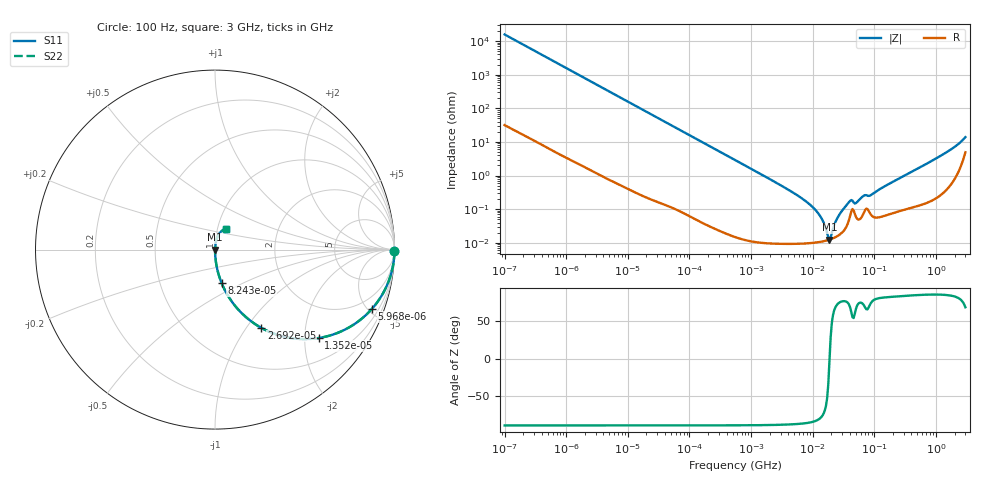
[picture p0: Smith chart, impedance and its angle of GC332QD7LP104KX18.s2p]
!Murata Part Number: GC332QD7LP104KX18
!These Parameters are Measured in Series Mode Connection
!Data Generated on Jun 10, 2025
!  o--ll--o
!Port1  Port2
!  o------o
!Operation Temp=25[degC], DC Bias Voltage=0[V]
!Freq. Start=100[Hz] Stop=3[GHz] 401[Steps]
# Hz S RI R 50
!Freq.(Hz) S11(Real) S11(Imag) S21(Real) S21(Imag) S12(Real) S12(Imag) S22(Real) S22(Imag)
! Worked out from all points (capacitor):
!   401 points, 100 Hz to 3 GHz, reference 50 ohm
!   read as one part in series: C = 101 nF near 109 Hz
!   lowest |Z| = 12.4 mohm at 18.68 MHz (marker M1)
!   series resonance near 18.76 MHz, so ESL is about 710 pH
!   S11 on the Smith chart (normalised r, x): 100 Hz: open; 5.968 kHz: 1.01, -5.29; 13.52 kHz: 1.01, -2.34; 26.92 kHz: 1.00, -1.18; 82.43 kHz: 1.00, -0.39; 3 GHz: 1.10, +0.26
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100  0.9999 -0.00637  5.34e-05 0.00637  5.34e-05 0.00637  0.9999 -0.00637
1788  0.9871 -0.1119  0.0129 0.1119  0.0129 0.1119  0.9871 -0.1119
5968  0.8744 -0.3302  0.1256 0.3302  0.1256 0.3302  0.8744 -0.3302
13520  0.5774 -0.4927  0.4226 0.4927  0.4226 0.4927  0.5774 -0.4927
26919  0.2575 -0.4358  0.7425 0.4358  0.7425 0.4358  0.2575 -0.4358
31977  0.1977 -0.3966  0.8023 0.3966  0.8023 0.3966  0.1977 -0.3966
82428  0.0364 -0.1854  0.9636 0.1854  0.9636 0.1854  0.0364 -0.1854
547723  0.000992 -0.029  0.999 0.029  0.999 0.029  0.000992 -0.029
4323298  0.000105 -0.00349  0.9999 0.00349  0.9999 0.00349  0.000105 -0.00349
9794414  0.0001 -0.00119  0.9999 0.00119  0.9999 0.00119  0.0001 -0.00119
1.382041e7  0.000108 -0.000532  0.9999 0.000532  0.9999 0.000532  0.000108 -0.000532
1.713898e7  0.000118 -0.000156  0.9999 0.000156  0.9999 0.000156  0.000118 -0.000156
1.867972e7  0.000124 -7.1e-06  0.9999 7.1e-06  0.9999 7.1e-06  0.000124 -7.1e-06
2.035898e7  0.000131 0.000142  0.9999 -0.000142  0.9999 -0.000142  0.000131 0.000142
2.635803e7  0.000168 0.000615  0.9998 -0.000615  0.9998 -0.000615  0.000168 0.000615
3.882828e7  0.000485 0.00156  0.9995 -0.00156  0.9995 -0.00156  0.000485 0.00156
5.026954e7  0.000592 0.00139  0.9994 -0.00139  0.9994 -0.00139  0.000592 0.00139
6.794454e7  0.000808 0.00241  0.9992 -0.00241  0.9992 -0.00241  0.000808 0.00241
8.79653e7  0.000691 0.00254  0.9993 -0.00254  0.9993 -0.00254  0.000691 0.00254
1.751444e8  0.000737 0.00569  0.9993 -0.00569  0.9993 -0.00569  0.000737 0.00569
1.268426e9  0.00457 0.0411  0.9954 -0.0411  0.9954 -0.0411  0.00457 0.0411
3e9  0.0614 0.1162  0.9386 -0.1162  0.9386 -0.1162  0.0614 0.1162
